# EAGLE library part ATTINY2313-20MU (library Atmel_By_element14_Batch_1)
Microcontroller
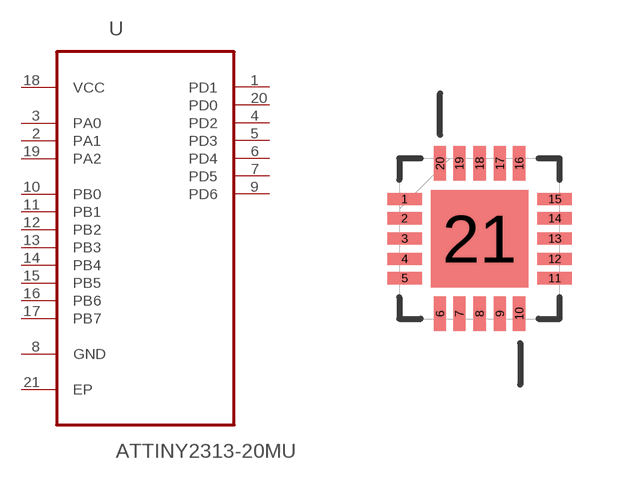
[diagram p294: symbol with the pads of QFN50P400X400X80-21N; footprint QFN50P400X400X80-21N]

Designator prefix U

## ATTINY2313-20MU (MPN: ATTINY2313-20MU; OC_FARNELL: 1748539; OC_NEWARK: 26R5646; PACKAGE: QFN-20; SUPPLIER: Atmel)  [QFN50P400X400X80-21N]
1  PD1
2  PA1
3  PA0
4  PD2
5  PD3
6  PD4
7  PD5
8  GND  pas
9  PD6
10  PB0
11  PB1
12  PB2
13  PB3
14  PB4
15  PB5
16  PB6
17  PB7
18  VCC  pwr
19  PA2
20  PD0
21  EP  pas

## Footprint QFN50P400X400X80-21N (pad centres in mm)
smd 0.864 x 0.305: 1 -1.88,0.991; 2 -1.88,0.508; 3 -1.88,0; 4 -1.88,-0.508; 5 -1.88,-0.991; 11 1.88,-0.991; 12 1.88,-0.508; 13 1.88,0; 14 1.88,0.508; 15 1.88,0.991
smd 0.305 x 0.864: 6 -0.991,-1.88; 7 -0.508,-1.88; 8 0,-1.88; 9 0.508,-1.88; 10 0.991,-1.88; 16 0.991,1.88; 17 0.508,1.88; 18 0,1.88; 19 -0.508,1.88; 20 -0.991,1.88
smd 2.438 x 2.438: 21 0,0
